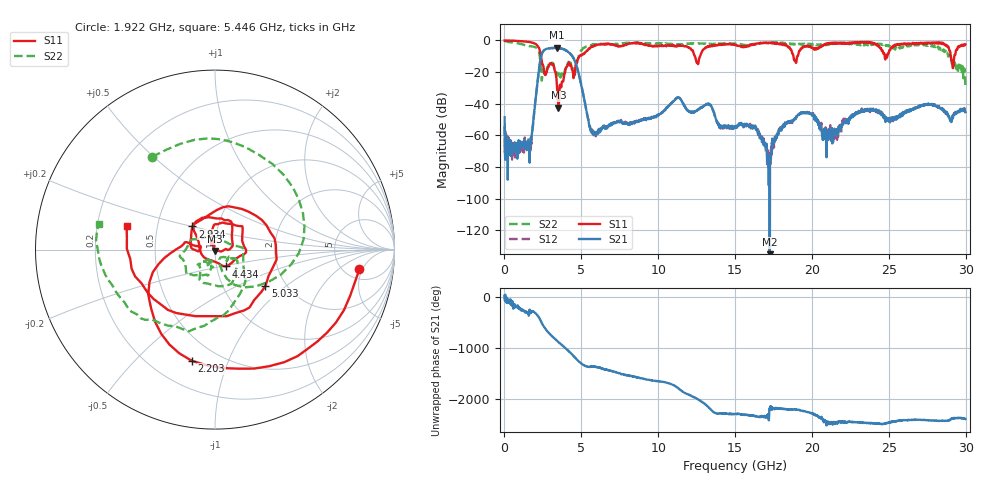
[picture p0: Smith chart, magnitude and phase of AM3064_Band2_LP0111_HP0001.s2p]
# Hz S DB R 50.0
!freq dBS11 angS11 dBS21 angS21 dBS12 angS12 dBS22 angS22
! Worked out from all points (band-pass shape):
!   1600 points, 10 MHz to 29.98 GHz, reference 50 ohm
!   highest |S21| = -4.60 dB at 3.403 GHz (marker M1); lowest = -199.0 dB at 17.25 GHz (marker M2)
!   |S21| within 3 dB of the highest: 2.473 GHz to 4.184 GHz (1.711 GHz wide, 51.4 % of centre)
!   lowest |S11| = -42.5 dB at 3.515 GHz (marker M3), VSWR 1.02, Z = 49.9 - j0.738 ohm
!   |S11| at or under -10 dB: 2.376 GHz to 4.881 GHz (2.506 GHz wide, 69 % of centre); 12.38 GHz to 12.72 GHz (341.6 MHz wide, 2.72 % of centre); 18.8 GHz to 19.05 GHz (252.1 MHz wide, 1.33 % of centre)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
!   |S22| runs from -28.8 to -0.2 dB; largest |S21 - S12| = 0.015
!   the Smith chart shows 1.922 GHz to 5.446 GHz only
!   S11 on the Smith chart (normalised r, x): 1.922 GHz: 6.84, -4.35; 2.203 GHz: 0.36, -0.75; 2.934 GHz: 0.75, +0.20; 4.434 GHz: 1.11, -0.21; 5.033 GHz: 1.58, -0.73; 5.446 GHz: 0.33, +0.12
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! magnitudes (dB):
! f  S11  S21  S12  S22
! 10 MHz  0.0  -48.6  -54.0  -0.2
! 1.547 GHz  -0.9  -65.5  -64.0  -3.5
! 1.922 GHz  -1.8  -46.2  -46.7  -4.1
! 2.203 GHz  -4.0  -22.1  -22.0  -6.1
! 2.934 GHz  -14.9  -5.0  -5.0  -13.7
! 3.403 GHz  -27.0  -4.6  -4.7  -21.0
! 3.515 GHz  -42.5  -4.7  -4.8  -21.9
! 4.434 GHz  -19.1  -10.2  -10.3  -17.4
! 5.015 GHz  -9.6  -29.0  -28.9  -6.4
! 5.033 GHz  -9.2  -29.7  -29.7  -6.0
! 5.446 GHz  -5.9  -49.5  -49.8  -3.6
! 10 GHz  -3.5  -47.5  -47.1  -2.0
! 11.31 GHz  -3.2  -36.2  -36.2  -2.7
! 15 GHz  -2.7  -54.0  -54.7  -2.0
! 16.3 GHz  -2.2  -54.6  -54.1  -2.2
! 17.25 GHz  -1.5  -199.0  -71.2  -1.2
! 18 GHz  -2.6  -57.0  -54.8  -1.8
! 19.99 GHz  -4.3  -46.7  -46.4  -2.2
! 20.82 GHz  -2.6  -55.7  -57.8  -2.5
! 25 GHz  -8.0  -49.9  -50.1  -3.1
! 28.31 GHz  -1.7  -42.6  -42.8  -4.6
! 29.98 GHz  -2.4  -45.4  -44.4  -28.8
